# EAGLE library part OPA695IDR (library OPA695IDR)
High Speed Operational Amplifiers Ultra-Wideband Curre nt Feedback Source: Datasheet
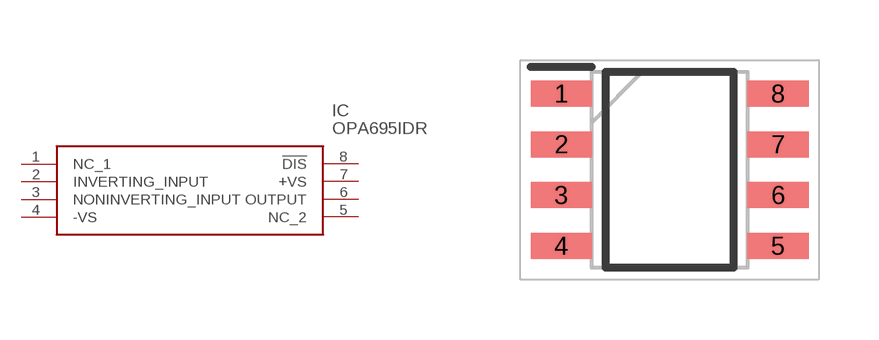
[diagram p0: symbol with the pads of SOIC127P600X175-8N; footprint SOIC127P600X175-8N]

Designator prefix IC

## OPA695IDR (Description: High Speed Operational Amplifiers Ultra-Wideband Curre nt Feedback; Height: 1.75mm; Manufacturer_Name: Texas Instruments; Manufacturer_Part_Number: OPA695IDR; Mouser_Part_Number: 595-OPA695IDR; Mouser_Price-Stock: https://www.mouser.co.uk/ProductDetail/Texas-Instruments/OPA695IDR?qs=wgAEGBTxy7loIslyoQGyeQ%3D%3D)  [SOIC127P600X175-8N]
1  NC_1
2  INVERTING_INPUT
3  NONINVERTING_INPUT
4  -VS
5  NC_2
6  OUTPUT
7  +VS
8  !DIS

## Footprint SOIC127P600X175-8N (pad centres in mm)
(D0008A_H=1.75
smd 1.528 x 0.65: 1 -2.711,1.905; 2 -2.711,0.635; 3 -2.711,-0.635; 4 -2.711,-1.905; 5 2.711,-1.905; 6 2.711,-0.635; 7 2.711,0.635; 8 2.711,1.905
